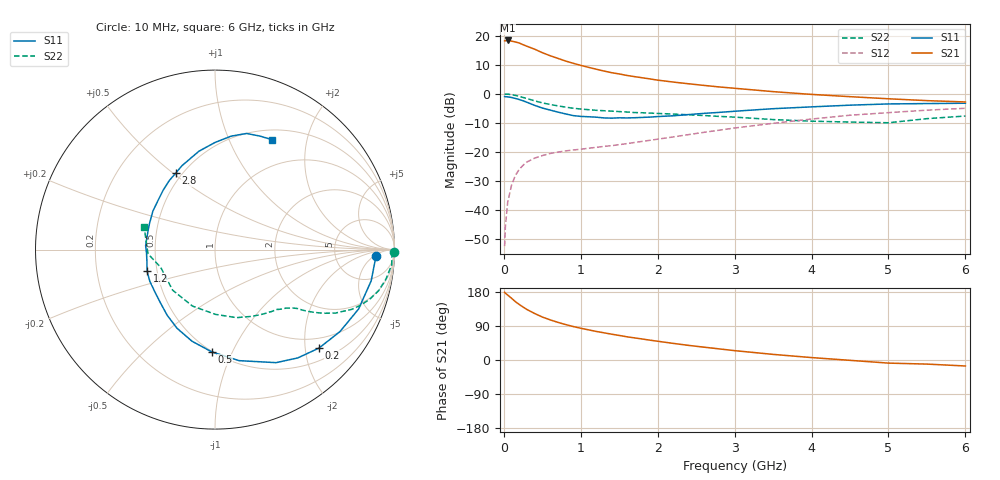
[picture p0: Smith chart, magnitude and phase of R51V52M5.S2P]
! SIEMENS Small Signal Semiconductors
! BFR183
! Si NPN RF Bipolar Junction Transistor in SOT23
! VCE = 1.5 V  IC = 2.5 mA
! Common Emitter S-Parameters:  May  1996
# GHz  S  MA  R  50
!  f  S11  S21  S12  S22
! GHz  MAG  ANG  MAG  ANG  MAG  ANG  MAG  ANG
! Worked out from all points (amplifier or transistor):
!   36 points, 10 MHz to 6 GHz, reference 50 ohm
!   highest |S21| = 18.4 dB at 50 MHz (marker M1)
!   |S21| within 3 dB of that: start of sweep to 400 MHz
!   unconditionally stable (mu >= 1): 1.283 GHz to 2.876 GHz
!   at 250 MHz: K = 0.27, MSG = 20.7 dB, |S12| = -24.6 dB
!   at 1.4 GHz: K = 1.05, MAG = 11.2 dB, |S12| = -17.8 dB
!   at 6 GHz: K = 0.92, MSG = 1.1 dB, |S12| = -5.0 dB
!   S11 on the Smith chart (normalised r, x): 10 MHz: 16, -6; 200 MHz: 0.76, -2.30; 500 MHz: 0.50, -0.84; 1.2 GHz: 0.44, -0.12; 2.8 GHz: 0.46, +0.51; 6 GHz: 0.62, +1.45
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0.01  0.8971 -2.4  8.145 178.6  0.0024 88.4  0.9948 -0.9
0.02  0.8931 -4.5  8.167 176.5  0.0052 85.6  0.9865 -1.9
0.05  0.8875 -11.3  8.279 171.3  0.0136 83.3  0.9885 -4.9
0.1  0.8658 -22.5  8.061 163.0  0.0268 77.8  0.9671 -9.7
0.15  0.8325 -33.3  7.798 154.0  0.0396 71.8  0.9401 -14.1
0.2  0.7981 -43.4  7.489 146.6  0.0502 67.0  0.9055 -17.8
0.3  0.716 -61.6  6.585 133.3  0.0673 59.2  0.8316 -23.6
0.4  0.6333 -77.7  5.861 122.8  0.0784 53.4  0.7582 -27.8
0.5  0.5702 -91.8  5.104 113.4  0.0867 49.2  0.699 -30.5
0.6  0.5263 -104.1  4.533 106.1  0.0942 46.7  0.657 -32.2
0.7  0.4869 -115.7  4.083 99.5  0.0994 45.1  0.6218 -33.6
0.8  0.4522 -126.2  3.675 93.7  0.1042 44.2  0.5916 -34.7
0.9  0.4228 -136.6  3.358 88.4  0.1081 44.4  0.5656 -35.5
1.1  0.4036 -154.3  2.856 79.6  0.116 45.0  0.5337 -37.6
1.2  0.397 -162.6  2.654 75.4  0.12 45.1  0.5213 -38.7
1.6  0.3852 169.8  2.07 61.2  0.1392 48.3  0.4867 -43.2
2.2  0.4187 139.5  1.595 43.9  0.1814 52.0  0.4493 -52.9
2.8  0.4797 117.0  1.313 29.3  0.2371 51.2  0.4092 -66.5
3.5  0.5553 99.3  1.091 14.8  0.3112 45.7  0.3609 -89.6
4.5  0.6385 81.9  0.894 -0.9  0.4286 33.7  0.3269 -136.2
5.5  0.68 68.5  0.764 -10.8  0.5237 19.9  0.3743 -176.4
6  0.6895 62.8  0.725 -15.8  0.5644 11.1  0.4152 162.1
